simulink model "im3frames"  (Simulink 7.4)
settings: Solver=ode45  StartTime=0.0  StopTime=2.0  MaxStep=1e-4  RelTol=1e-3  AbsTol=1e-3
libraries: simulink x4

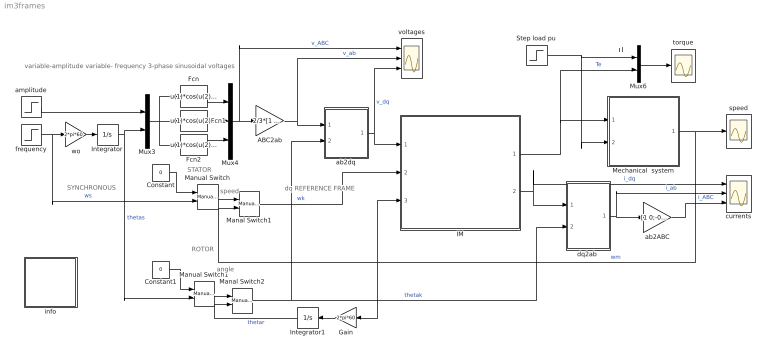
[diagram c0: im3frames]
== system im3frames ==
  note: dq REFERENCE FRAME
  note: STATOR
  note: SYNCHRONOUS
  note: ROTOR
  note: variable-amplitude variable- frequency 3-phase sinusoidal voltages
  note: Tl
  note: speed
  note: angle
  ABC2ab : Gain  Gain=2/3*[1 -0.5 -0.5;0 sqrt(3)/2 -sqrt(3)/2]  Multiplication=Matrix(K*u)  ParameterDataType=sfix(16)  ParameterScaling=2^0  OutDataType=sfix(16)  OutScaling=2^0
  Constant : Constant  Value=0  OutDataType=sfix(16)  OutScaling=2^0
  Constant1 : Constant  Value=0  OutDataType=sfix(16)  OutScaling=2^0
  Fcn : Fcn  Expr=u(1)*cos(u(2)+pi/6)
  Fcn1 : Fcn  Expr=u(1)*cos(u(2)-2*pi/3+pi/6)
  Fcn2 : Fcn  Expr=u(1)*cos(u(2)+2*pi/3+pi/6)
  Gain : Gain  Gain=2*pi*60  ParameterDataType=sfix(16)  ParameterScaling=2^0  OutDataType=sfix(16)  OutScaling=2^0
  IM : Subsystem  mask{Rs=0.01, Rr=0.02, Lsl=0.10, Lrl=0.10, Lm=4.5, wo=2*pi*60}
      mask prompts: Rs "Stator resistance [pu]"; Rr "Rotor resistance [pu]"; Lsl "Stator leakage inductance [pu]"; Lrl "Rotor leakage inductance [pu]"; Lm "Magnetizing inductance [pu]"; wo "Base frequency [rad/s]"
      mask help: Induction machine dynamic representation in selected reference frame
  Integrator : Integrator
  Integrator1 : Integrator
  Manal Switch1 : simulink/Signal Routing/Manual Switch  SystemSampleTime=-1  sw=1  action=0  varsize=off
  Manal Switch2 : simulink/Signal Routing/Manual Switch  SystemSampleTime=-1  sw=1  action=0  varsize=off
  Manual Switch : simulink/Signal Routing/Manual Switch  SystemSampleTime=-1  sw=0  action=0  varsize=off
  Manual Switch1 : simulink/Signal Routing/Manual Switch  SystemSampleTime=-1  sw=0  action=0  varsize=off
  Mechanical  system : Subsystem  mask{H=0.3, Bm=1e-5}
      mask prompts: H "Inertia constant [s]"; Bm "Torque-speed coefficient"
      mask help: Mechanical system represented by an inertia and a damping term
  Mux3 : Mux  Inputs=2
  Mux4 : Mux  Inputs=3
  Mux6 : Mux  Inputs=2
  Step load pu : Step  Time=1.7  After=1.0  SampleTime=0
  ab2ABC : Gain  Gain=[1 0;-0.5 sqrt(3)/2;-0.5 -sqrt(3)/2]  Multiplication=Matrix(K*u)  ParameterDataType=sfix(16)  ParameterScaling=2^0  OutDataType=sfix(16)  OutScaling=2^0
  ab2dq : Subsystem
  amplitude : Step  Time=1.4  Before=1  After=5/6  SampleTime=0
  currents : Scope  NumInputPorts=3
  "dq2ab " : Subsystem
  frequency : Step  Time=1.4  Before=1  After=5/6  SampleTime=0
  info : Subsystem
  speed : Scope
  torque : Scope
  voltages : Scope  NumInputPorts=3
  wo : Gain  Gain=2*pi*60  ParameterDataType=sfix(16)  ParameterScaling=2^0  OutDataType=sfix(16)  OutScaling=2^0
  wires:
  IM/2(is) -> "dq2ab "/1(dq), currents/1  "i_dq"
  Mux6/1 -> torque/1
  Step load pu/1 -> Mux6/1, Mechanical  system/2(Tl)
  IM/1(Te) -> Mux6/2, Mechanical  system/1(Te)  "Te"
  Mechanical  system/1(wm) -> speed/1, IM/3(wm), Manal Switch1/2, Gain/1  "wm"
  ab2dq/1(dq) -> IM/1(vs), voltages/3  "v_dq"
  frequency/1 -> wo/1, Manual Switch/2  "ws"
  Mux4/1 -> ABC2ab/1, voltages/1  "v_ABC"
  Fcn/1 -> Mux4/1
  Fcn1/1 -> Mux4/2
  Fcn2/1 -> Mux4/3
  ABC2ab/1 -> ab2dq/1(ab), voltages/2  "v_ab"
  wo/1 -> Integrator/1
  Integrator/1 -> Mux3/2, Manual Switch1/2  "thetas"
  amplitude/1 -> Mux3/1
  Mux3/1 -> Fcn1/1, Fcn/1, Fcn2/1
  Constant/1 -> Manual Switch/1
  Manual Switch/1 -> Manal Switch1/1
  Manal Switch1/1 -> IM/2(wk)  "wk"
  Gain/1 -> Integrator1/1
  Manual Switch1/1 -> Manal Switch2/1
  Manal Switch2/1 -> ab2dq/2(thetak), "dq2ab "/2(thetak)  "thetak"
  Constant1/1 -> Manual Switch1/1
  Integrator1/1 -> Manal Switch2/2  "thetar"
  "dq2ab "/1(ab) -> ab2ABC/1, currents/2  "i_ab"
  ab2ABC/1 -> currents/3  "i_ABC"

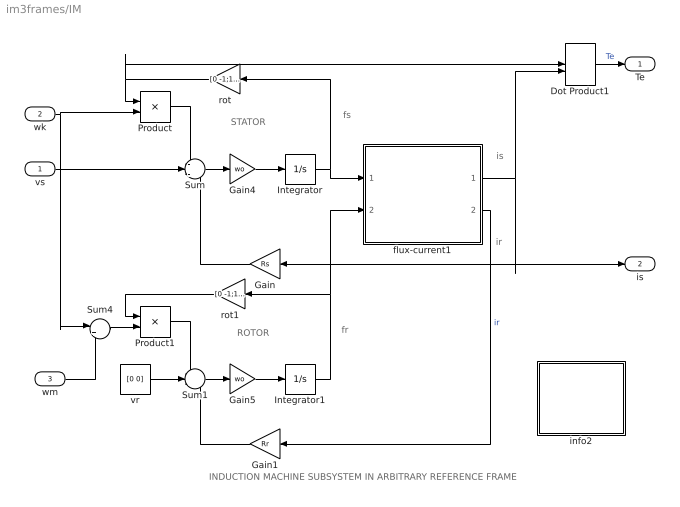
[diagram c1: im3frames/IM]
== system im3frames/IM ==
  note: ROTOR
  note: STATOR
  note: fs
  note: fr
  note: is
  note: INDUCTION MACHINE SUBSYSTEM IN ARBITRARY REFERENCE FRAME
  note: ir
  vs : Inport  OutDataType=sfix(16)  OutScaling=2^0
  wk : Inport  Port=2  OutDataType=sfix(16)  OutScaling=2^0
  wm : Inport  Port=3  OutDataType=sfix(16)  OutScaling=2^0
  Dot Product1 : DotProduct  OutDataType=fixdt(1, 16)  OutScaling=2^-10
  Gain : Gain  Gain=Rs  ParameterDataType=sfix(16)  ParameterScaling=2^0  OutDataType=sfix(16)  OutScaling=2^0
  Gain1 : Gain  Gain=Rr  ParameterDataType=sfix(16)  ParameterScaling=2^0  OutDataType=sfix(16)  OutScaling=2^0
  Gain4 : Gain  Gain=wo  ParameterDataType=sfix(16)  ParameterScaling=2^0  OutDataType=sfix(16)  OutScaling=2^0
  Gain5 : Gain  Gain=wo  ParameterDataType=sfix(16)  ParameterScaling=2^0  OutDataType=sfix(16)  OutScaling=2^0
  Integrator : Integrator  InitialCondition=[0 0]
  Integrator1 : Integrator  InitialCondition=[0 0]
  Product : Product  OutDataType=sfix(16)  OutScaling=2^0
  Product1 : Product  OutDataType=sfix(16)  OutScaling=2^0
  Sum : Sum  Inputs=-+-  OutDataType=sfix(16)  OutScaling=2^0
  Sum1 : Sum  Inputs=-+-  OutDataType=sfix(16)  OutScaling=2^0
  Sum4 : Sum  Inputs=|+-  OutDataType=sfix(16)  OutScaling=2^0
  flux-current1 : Subsystem
  info2 : Subsystem
  rot : Gain  Gain=[0 -1;1 0]  Multiplication=Matrix(K*u)  ParameterDataType=sfix(16)  ParameterScaling=2^0  OutDataType=sfix(16)  OutScaling=2^0
  rot1 : Gain  Gain=[0 -1;1 0]  Multiplication=Matrix(K*u)  ParameterDataType=sfix(16)  ParameterScaling=2^0  OutDataType=sfix(16)  OutScaling=2^0
  vr : Constant  Value=[0 0]  OutDataType=sfix(16)  OutScaling=2^0
  Te : Outport
  is : Outport  Port=2
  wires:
  Gain/1 -> Sum/3
  vr/1 -> Sum1/2
  Gain1/1 -> Sum1/3
  flux-current1/2(ir) -> Gain1/1  "ir"
  Integrator/1 -> flux-current1/1(fs), rot/1
  Integrator1/1 -> flux-current1/2(fr), rot1/1
  Product1/1 -> Sum1/1
  rot1/1 -> Product1/1
  Product/1 -> Sum/1
  rot/1 -> Product/1, Dot Product1/1
  Sum4/1 -> Product1/2
  Sum/1 -> Gain4/1
  Gain4/1 -> Integrator/1
  Sum1/1 -> Gain5/1
  Gain5/1 -> Integrator1/1
  flux-current1/1(is) -> Gain/1, is/1, Dot Product1/2
  Dot Product1/1 -> Te/1  "Te"
  vs/1 -> Sum/2
  wk/1 -> Product/2, Sum4/1
  wm/1 -> Sum4/2

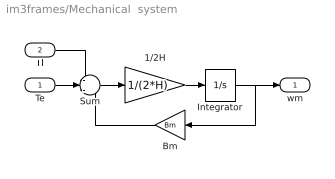
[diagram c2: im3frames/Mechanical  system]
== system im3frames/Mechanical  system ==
  Te : Inport  OutDataType=sfix(16)  OutScaling=2^0
  Tl : Inport  Port=2  OutDataType=sfix(16)  OutScaling=2^0
  1/2H : Gain  Gain=1/(2*H)  ParameterDataType=sfix(16)  ParameterScaling=2^0  OutDataType=sfix(16)  OutScaling=2^0
  Bm : Gain  Gain=Bm  ParameterDataType=sfix(16)  ParameterScaling=2^0  OutDataType=sfix(16)  OutScaling=2^0
  Integrator : Integrator
  Sum : Sum  Inputs=-+-  OutDataType=sfix(16)  OutScaling=2^0
  wm : Outport
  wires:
  1/2H/1 -> Integrator/1
  Sum/1 -> 1/2H/1
  Bm/1 -> Sum/3
  Integrator/1 -> Bm/1, wm/1
  Te/1 -> Sum/2
  Tl/1 -> Sum/1

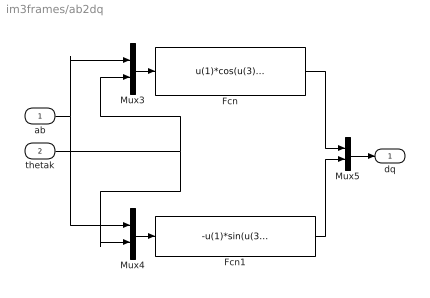
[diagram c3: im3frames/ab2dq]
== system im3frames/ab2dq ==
  ab : Inport  OutDataType=sfix(16)  OutScaling=2^0
  thetak : Inport  Port=2  OutDataType=sfix(16)  OutScaling=2^0
  Fcn : Fcn  Expr=u(1)*cos(u(3))+u(2)*sin(u(3))
  Fcn1 : Fcn  Expr=-u(1)*sin(u(3))+u(2)*cos(u(3))
  Mux3 : Mux  Inputs=2
  Mux4 : Mux  Inputs=2
  Mux5 : Mux  Inputs=2
  dq : Outport
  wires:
  Mux3/1 -> Fcn/1
  Mux4/1 -> Fcn1/1
  ab/1 -> Mux3/1, Mux4/1
  thetak/1 -> Mux3/2, Mux4/2
  Fcn1/1 -> Mux5/2
  Fcn/1 -> Mux5/1
  Mux5/1 -> dq/1

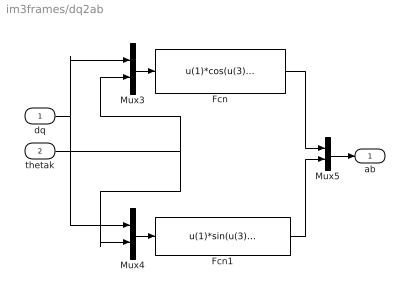
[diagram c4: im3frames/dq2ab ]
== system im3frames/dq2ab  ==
  dq : Inport  OutDataType=sfix(16)  OutScaling=2^0
  thetak : Inport  Port=2  OutDataType=sfix(16)  OutScaling=2^0
  Fcn : Fcn  Expr=u(1)*cos(u(3))-u(2)*sin(u(3))
  Fcn1 : Fcn  Expr=u(1)*sin(u(3))+u(2)*cos(u(3))
  Mux3 : Mux  Inputs=2
  Mux4 : Mux  Inputs=2
  Mux5 : Mux  Inputs=2
  ab : Outport
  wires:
  Mux5/1 -> ab/1
  Fcn/1 -> Mux5/1
  Fcn1/1 -> Mux5/2
  thetak/1 -> Mux4/2, Mux3/2
  dq/1 -> Mux4/1, Mux3/1
  Mux4/1 -> Fcn1/1
  Mux3/1 -> Fcn/1

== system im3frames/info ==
  note: A selection of one of three common reference frames is obtained by clicking the manual switches: a)Stator frame where wk=0 and thetak=0 indicated in cyan color. b)Synchronous frame where wk=ws and thetak = wo int(ws) indicated in red. c)Rotor frame where wk=wm and thetak = wo int(wm) in green. (wo is the base frequency 2 pi fo [rad/s] where fo = 60 Hz) Both upper and lower pair of switches must be in the same up or down positions. The induction machine is modeled in vectorized form in conformity with state vector formulation. The parameters describing the electromechanical system are expressed in per unit. The three-phase sinusoidal excitation can be adjusted in both amplitude and frequency. In this simulation, the system is assumed to be initially inert so that all the initial conditions are zero. The motor is started at no load at rated voltage and frequency. After reaching steady-state conditions, the input voltage is suddenly reduced by a factor of 5/6 in amplitude and frequency and soon after full load is applied as a step function. The voltages and currents can be observed on the scopes in both stator and rotating frames. Note that, in steady-state, the stator currents show up at stator frequency ws in the stator frame, as dc quantities in the synchronous frame, and at slip frequency (ws-wm) in the rotor frame. The torque and speed time evolutions do not depend on the choice of reference frame.
  note: Running of an Induction Motor Modeled in Three Reference Frames under Three-Phase Sinusoidal Excitation

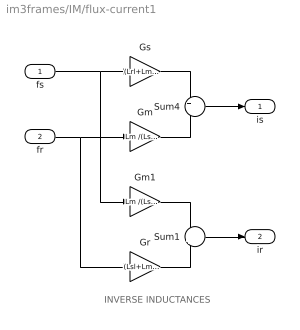
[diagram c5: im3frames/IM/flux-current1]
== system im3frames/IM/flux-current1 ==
  note: INVERSE INDUCTANCES
  fs : Inport  OutDataType=sfix(16)  OutScaling=2^0
  fr : Inport  Port=2  OutDataType=sfix(16)  OutScaling=2^0
  Gm : Gain  Gain=Lm /(Lsl*Lrl+Lsl*Lm+Lrl*Lm)  ParameterDataType=sfix(16)  ParameterScaling=2^0  OutDataType=sfix(16)  OutScaling=2^0
  Gm1 : Gain  Gain=Lm /(Lsl*Lrl+Lsl*Lm+Lrl*Lm)  ParameterDataType=sfix(16)  ParameterScaling=2^0  OutDataType=sfix(16)  OutScaling=2^0
  Gr : Gain  Gain=(Lsl+Lm )/(Lsl*Lrl+Lsl*Lm+Lrl*Lm)  ParameterDataType=sfix(16)  ParameterScaling=2^0  OutDataType=sfix(16)  OutScaling=2^0
  Gs : Gain  Gain=(Lrl+Lm) /(Lsl*Lrl+Lsl*Lm+Lrl*Lm)  ParameterDataType=sfix(16)  ParameterScaling=2^0  OutDataType=sfix(16)  OutScaling=2^0
  Sum1 : Sum  Inputs=-+  OutDataType=sfix(16)  OutScaling=2^0
  Sum4 : Sum  Inputs=+-  OutDataType=sfix(16)  OutScaling=2^0
  is : Outport
  ir : Outport  Port=2
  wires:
  fs/1 -> Gs/1, Gm1/1
  Gs/1 -> Sum4/1
  fr/1 -> Gm/1, Gr/1
  Gm/1 -> Sum4/2
  Sum4/1 -> is/1
  Gm1/1 -> Sum1/1
  Gr/1 -> Sum1/2
  Sum1/1 -> ir/1

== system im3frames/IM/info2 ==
  note: Synchronous machine transients under shortcircuit
  note: This demonstration illustrates the dynamics of a synchronous generator, initially at no load, following a three-phase short circuit at the terminals.
